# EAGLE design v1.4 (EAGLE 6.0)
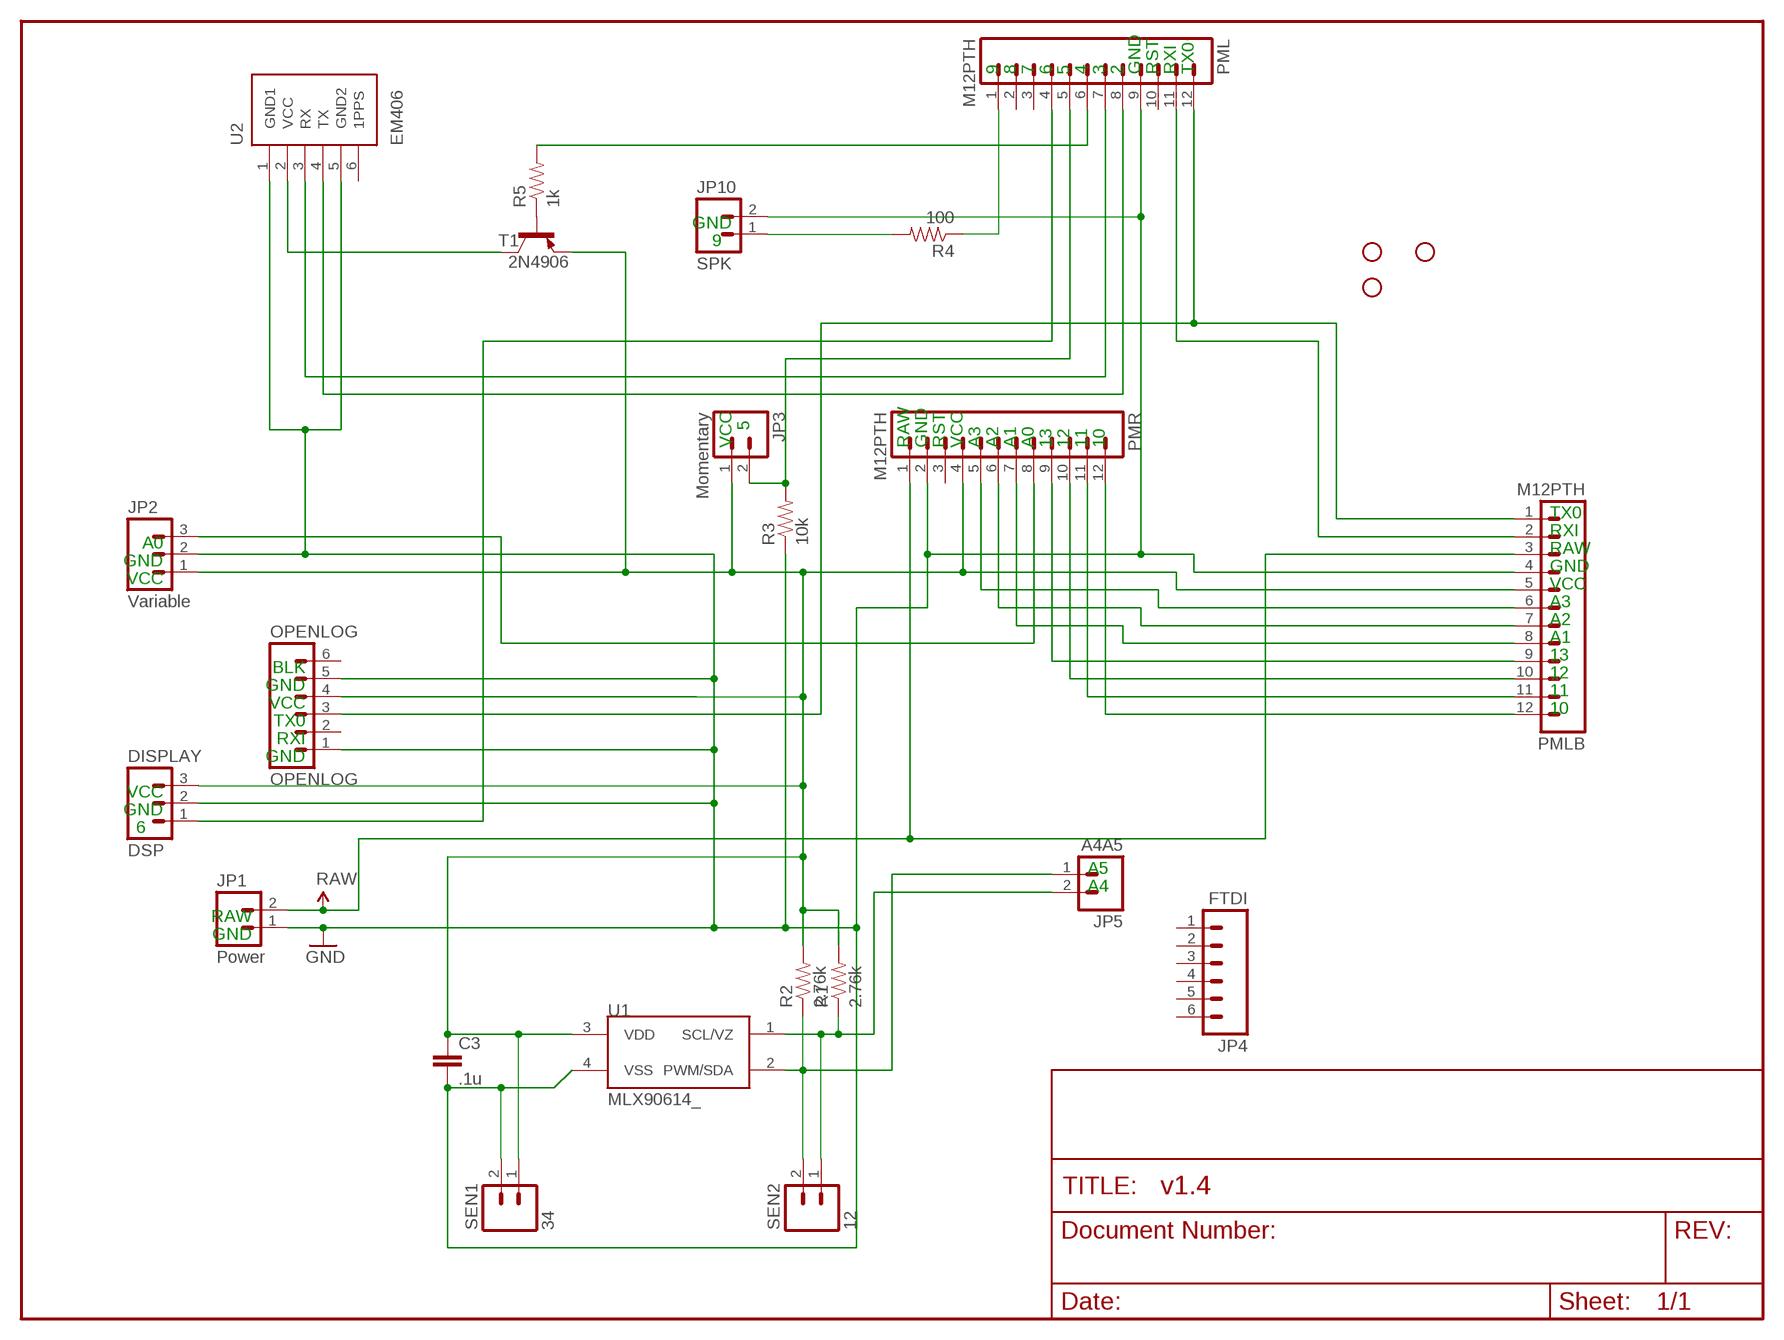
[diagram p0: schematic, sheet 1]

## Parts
2N4906  T1  2N3906-PNP-TO92-EBC  [TO92-EBC]
C3  .1u  CAPPTH1  [CAP-PTH-5MM]
DISPLAY  DSP  M03SCREW_LOCK  [SCREWTERMINAL-3.5MM-3_LOCK.007S]
JP1  Power  M02JST-PTH-2  [JST-2-PTH]
JP2  Variable  M03SCREW_LOCK  [SCREWTERMINAL-3.5MM-3_LOCK.007S]
JP3  Momentary  M02JST-PTH-2  [JST-2-PTH]
JP4  FTDI  M06SIP  [1X06]
JP5  A4A5  M02PTH  [1X02]
JP6  STAND-OFFTIGHT  [STAND-OFF-TIGHT]
JP7  STAND-OFFTIGHT  [STAND-OFF-TIGHT]
JP8  STAND-OFFTIGHT  [STAND-OFF-TIGHT]
JP10  SPK  M02JST-PTH-2  [JST-2-PTH]
OPENLOG  OPENLOG  M06LOCK  [1X06_LOCK]
PML  M12PTH  [1X12]
PMLB  M12PTH  [1X12]
PMR  M12PTH  [1X12]
R1  2.76k  RESISTORPTH-1/4W  [AXIAL-0.4]
R2  2.76k  RESISTORPTH-1/4W  [AXIAL-0.4]
R3  10k  RESISTORPTH-1/4W  [AXIAL-0.4]
R4  100  RESISTORPTH-1/4W  [AXIAL-0.4]
R5  1k  RESISTORPTH-1/4W  [AXIAL-0.4]
SEN1  34  M02JST-PTH-2  [JST-2-PTH]
SEN2  12  M02JST-PTH-2  [JST-2-PTH]
U1  MLX90614_  [TO-39]
U2  EM406  [EM406]

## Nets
GND: C3.2 DISPLAY.2 JP1.1 JP2.2 JP10.2 OPENLOG.1 OPENLOG.5 PML.9 PMLB.4 PMR.2 R3.P$1 SEN1.2 U1.4(VSS) U2.1(GND1) U2.5(GND2)
N$1: JP10.1 R4.P$2
N$2: JP5.1 R2.P$1 SEN2.2 U1.2(PWM/SDA)
N$3: JP3.2 PML.5 R3.P$2
N$4: DISPLAY.1 PML.4
N$5: JP2.3 PMR.8
N$6: OPENLOG.3 PML.12 PMLB.1
N$8: PML.11 PMLB.2
N$9: PMLB.12 PMR.12
N$10: PMLB.11 PMR.11
N$11: PMLB.10 PMR.10
N$12: PMLB.9 PMR.9
N$13: PMLB.8 PMR.7
N$14: PMLB.7 PMR.6
N$15: PMLB.6 PMR.5
N$16: 2N4906.E C3.1 DISPLAY.3 JP2.1 JP3.1 OPENLOG.4 PMLB.5 PMR.4 R1.P$2 R2.P$2 SEN1.1 U1.3(VDD)
N$17: PML.1 R4.P$1
N$18: 2N4906.B R5.P$1
N$19: 2N4906.C U2.2(VCC)
N$20: PML.8 U2.4(TX)
N$21: PML.7 U2.3(RX)
N$22: PML.6 R5.P$2
SENSOR: JP5.2 R1.P$1 SEN2.1 U1.1(SCL/VZ)
VCC: JP1.2 PMLB.3 PMR.1 ; supply symbol labelled RAW
Unconnected: JP4.1 JP4.2 JP4.3 JP4.4 JP4.5 JP4.6 OPENLOG.2 OPENLOG.6 PML.2 PML.3 PML.10 PMR.3 U2.6(1PPS)

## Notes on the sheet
- 9 | 8 | 7 | 6 | 5 | 4 | 3 | 2 | GND | RST | RXI | TX0
- GND
- 9
- 5
- VCC | RAW | GND | RST | VCC | A3 | A2 | A1 | A0 | 13 | 12 | 11 | 10
- TX0
- A0 | RXI
- GND | RAW
- VCC | GND
- VCC
- A3
- A2
- A1
- BLK | 13
- GND | 12
- VCC | 11
- TX0 | 10
- RXI
- GND
- VCC
- GND
- 6
- A5
- A4
- RAW
- GND

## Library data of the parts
2N4906 = transistor-neu-to92:*-PNP-: PNP Transistror
C3 = SparkFun:CAP: Capacitor
DISPLAY JP2 = SparkFun:M03: Header 3 Standard 3-pin 0.1" header. Use with straight break away headers (SKU : PRT-00116), right angle break away headers (PRT-00553), swiss pins (PRT-00743), machine pins (PRT-00117), and female headers (PRT-00115). Molex polarized connector foot print use with SKU : PRT-08232 with associated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
JP1 JP3 JP5 JP10 SEN1 SEN2 = SparkFun:M02: Header 2
JP4 OPENLOG = SparkFun:M06: Header 6 Standard 6-pin 0.1" header. Use with straight break away headers (SKU : PRT-00116), right angle break away headers (PRT-00553), swiss pins (PRT-00743), machine pins (PRT-00117), and female headers (PRT-00115). Molex polarized connector foot print use with SKU : PRT-08094 with associated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
JP6-JP8 = SparkFun:STAND-OFF: Stand Off
PML PMLB PMR = SparkFun:M12: Header 12 Standard 12-pin 0.1" header. Use with straight break away headers (SKU : PRT-00116), right angle break away headers (PRT-00553), swiss pins (PRT-00743), machine pins (PRT-00117), and female headers (PRT-00115).
R1-R5 = SparkFun:RESISTOR: Resistor
U1 = SparkFun:MLX90614: Melexis IR Thermometer
U2 = SparkFun:EM406: EM406 Connector Proven layout and schematic for EM406 connector. Spark Fun Electronics SKU : GPS-00579

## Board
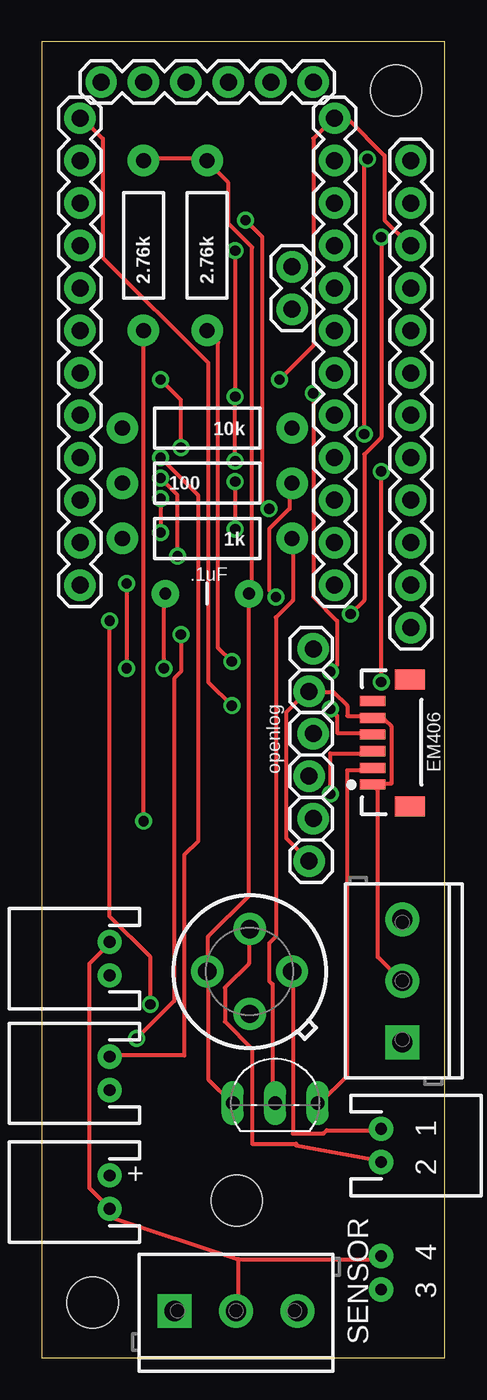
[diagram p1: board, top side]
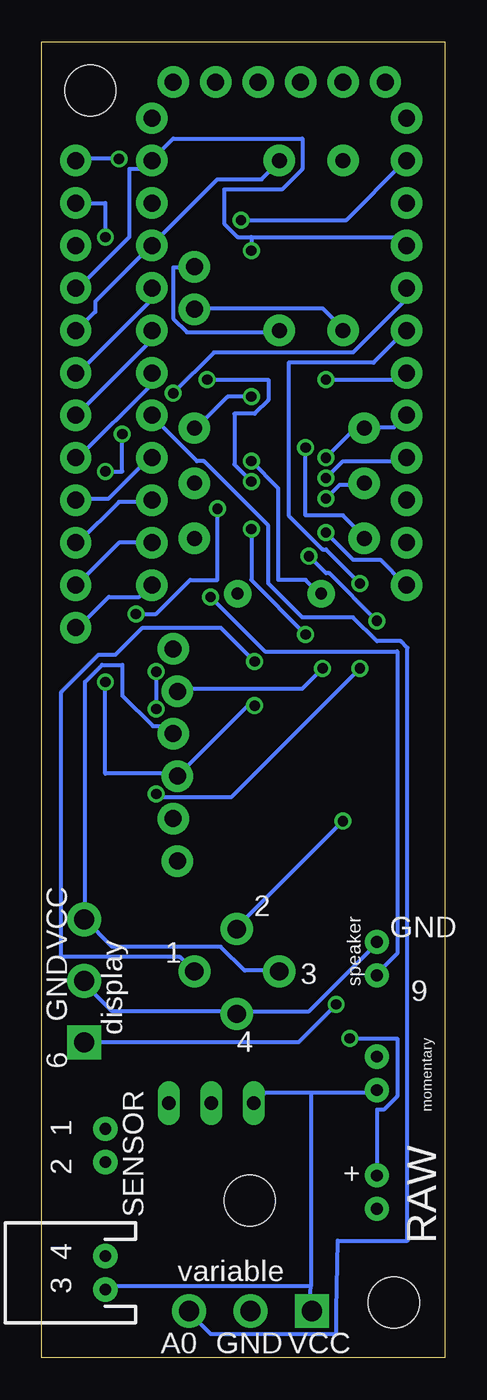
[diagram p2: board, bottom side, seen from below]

Size 24.13 x 78.74 mm. Coordinates in mm from the lower left corner, seen from the top.
Outline: 0,0 24.13,0 24.13,78.74 0,78.74 0,0
Copper layers (1*16): Top 0.035mm / dielectric 1.5mm / Bottom 0.035mm
Design rules: minimum track width 10mil, minimum drill 24mil, track to track 8mil, track to pad 8mil, pad to pad 8mil, via to via 8mil, smd to smd 8mil, copper to edge 40mil, drill to drill 8mil, minimum pad ring 10mil, minimum via ring 8mil, stop-mask expansion 4mil, vias tented up to drill 0mil, thermal gap 10mil

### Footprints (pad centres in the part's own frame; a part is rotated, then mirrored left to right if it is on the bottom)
TO92-EBC = drill 0.813 long: B 0,-1.27; C 2.54,-1.27; E -2.54,-1.27
CAP-PTH-5MM = drill 0.7 pad 1.651: 1 -2.5,0; 2 2.5,0
SCREWTERMINAL-3.5MM-3_LOCK.007S = drill 1.2 pad 2.032 square: 1 -0.178,0 | drill 1.2 pad 2.032: 2 3.5,0; 3 7.178,0
JST-2-PTH = drill 0.7 pad 1.448: 1 -1,0; 2 1,0
1X06 = drill 1.016 pad 1.88: 1 0,0; 2 2.54,0; 3 5.08,0; 4 7.62,0; 5 10.16,0; 6 12.7,0
1X02 = drill 1.016 pad 1.88: 1 0,0; 2 2.54,0
STAND-OFF-TIGHT = hole 3.048: 0,0
1X06_LOCK = drill 1.016 pad 1.88: 1 0,0; 2 2.54,-0.254; 3 5.08,0; 4 7.62,-0.254; 5 10.16,0; 6 12.7,-0.254
1X12 = drill 1.016 pad 1.88: 1 0,0; 2 2.54,0; 3 5.08,0; 4 7.62,0; 5 10.16,0; 6 12.7,0; 7 15.24,0; 8 17.78,0; 9 20.32,0; 10 22.86,0; 11 25.4,0; 12 27.94,0
AXIAL-0.4 = drill 0.9 pad 1.88: P$1 -5.08,0; P$2 5.08,0
TO-39 = drill 1.1 pad 1.93: 1 2.54,0; 2 0,2.54; 3 -2.54,0; 4 0,-2.54
EM406 = smd 0.6 x 1.55: 1 0,0; 2 1,0; 3 2,0; 4 3,0; 5 4,0; 6 5,0 | smd 1.2 x 1.8: P$1 -1.3,-2.225; P$2 6.3,-2.225

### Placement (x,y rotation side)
2N4906  13.97,16.51 0 top
C3  9.91,45.72 180 top
DISPLAY  21.59,19.05 90 top
JP1  4.06,9.91 90 top
JP2  8.13,2.79 0 top
JP3  4.06,17.02 90 top
JP4  16.26,76.33 180 top
JP5  14.99,62.74 90 top
JP6  3.05,3.3 0 top
JP7  21.21,75.82 0 top
JP8  11.68,9.4 90 top
JP10  4.06,23.88 90 top
OPENLOG  16,29.72 90 top
PML  2.29,46.23 90 top
PMLB  22.1,71.63 270 top
PMR  17.53,74.17 270 top
R1  9.91,66.55 90 top
R2  6.1,66.55 90 top
R3  9.91,55.63 180 top
R4  9.91,52.32 0 top
R5  9.91,49.02 180 top
SEN1  20.32,5.08 90 bottom
SEN2  20.32,12.7 270 top
U1  12.45,23.11 0 top
U2  19.81,34.29 90 top

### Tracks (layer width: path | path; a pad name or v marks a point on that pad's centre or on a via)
GND  (via drill 0.61)
  Top 0.254: v11.58,66.24 v11.58,57.51 v11.58,53.65 | v7.32,41.25 7.32,45.72 C3.2 | OPENLOG.1 14.63,31.09 14.63,38.61 15.85,39.83 OPENLOG.5 16.05,39.83 17.48,39.83 18.29,39.01 18.29,38.41 19.71,38.41 U2.5 19.91,38.2 20.52,38.2 20.93,37.8 20.93,34.34 19.91,34.34 U2.1 19.91,34.14 20.12,33.93 20.12,23.98 21.54,22.55 DISPLAY.2 | JP10.2 4.06,24.79 2.85,23.57 2.85,10.16 4.06,8.94 JP1.1 4.06,8.43 11.79,5.89 | 11.79,5.89 20.32,5.89 SEN1.2 | 11.79,5.89 11.79,2.85 JP2.2
  Bottom 0.254: 11.58,67.06 12.39,67.06 13.21,67.87 13.21,69.9 9.75,69.9 8.53,71.12 8.53,72.95 16.26,72.95 17.48,71.73 PMR.2 17.68,71.53 18.09,71.12 18.9,71.12 18.9,67.06 21.95,64.01 PMLB.4 | 11.58,67.06 2.85,67.06 2.44,66.65 PML.9 | v11.58,57.51 13.01,57.51 14.83,55.68 R3.P$1 | 11.58,67.06 v11.58,66.24 | v7.32,41.25 8.53,40.03 15.85,40.03 OPENLOG.5 | JP10.2 4.06,24.79 8.13,20.73 12.39,20.73 U1.4 12.6,20.73 19.91,20.73 21.54,22.35 DISPLAY.2 | v11.58,53.65 9.96,52.02 9.96,46.53 8.33,46.53 7.52,45.72 C3.2
N$1  (via drill 0.61)
  Top 0.254: v14.02,45.52 13.61,45.92 13.61,49.58 14.83,50.8 14.83,52.22 R4.P$2
  Bottom 0.254: v14.02,45.52 10.77,42.27 2.85,42.27 2.85,24.18 4.06,22.96 JP10.1
N$2  (via drill 0.61)
  Top 0.254: v6.1,32.11 R2.P$1 | SEN2.2 20.32,11.79 15.24,12.7 15.24,12.8 12.6,12.8 12.6,18.49 10.97,20.12 10.97,22.15 12.39,23.57 12.39,25.6 U1.2
  Bottom 0.254: R2.P$1 6.1,61.57 7.32,62.79 14.83,62.79 JP5.1 | v6.1,32.11 12.39,25.81 U1.2
N$3  (via drill 0.61)
  Top 0.254: v7.11,53.85 9.35,51.61 9.35,30.89 8.53,30.07 8.53,18.09 4.06,18.09 JP3.2
  Bottom 0.254: v7.11,53.85 5.49,55.47 4.88,55.47 R3.P$2 4.67,55.68 3.05,55.68 2.44,56.29 PML.5
N$4  (via drill 0.61)
  Top 0.254: v7.11,52.63 8.13,51.61 v8.13,47.95 | v4.06,44.09 4.06,26.42 6.5,23.98 v6.5,21.13
  Bottom 0.254: v7.11,52.63 6.1,53.65 2.64,53.65 2.44,53.85 PML.4 | v8.13,47.95 7.11,46.94 6.91,46.94 v4.06,44.09 | v6.5,21.13 8.74,18.9 21.54,18.9 DISPLAY.1
N$5
  Bottom 0.254: PMR.8 17.48,56.29 14.83,53.65 14.43,53.65 10.57,49.78 10.57,46.33 8.53,44.3 5.49,44.3 4.06,42.88 2.64,42.88 2.23,42.47 2.23,7.01 6.4,7.01 6.5,2.85 6.5,1.42 14.02,1.42 15.24,2.64 JP2.3
N$6  (via drill 0.61)
  Top 0.254: v11.38,39.01 9.96,40.44 9.96,59.54 3.66,65.84 3.66,72.95 2.44,74.17 PML.12 | v19.51,71.73 19.3,71.53 v19.3,55.27 | v20.32,40.44 v20.32,53.03
  Bottom 0.254: v11.38,39.01 11.79,39.01 OPENLOG.3 16.05,34.95 20.32,34.95 v20.32,40.44 | v19.51,71.73 21.95,71.73 PMLB.1 | v19.3,55.27 19.3,53.03 v20.32,53.03
N$8  (via drill 0.61)
  Top 0.254: v12.19,68.07 13.21,67.06 13.21,51.21 v13.61,50.8 | v18.49,44.5 19.3,45.31 19.3,54.05 20.32,55.07 v20.32,67.06
  Bottom 0.254: v12.19,68.07 5.89,68.07 2.44,71.53 PML.11 | v13.61,50.8 13.61,46.53 15.24,46.53 17.27,44.5 v18.49,44.5 | v20.32,67.06 20.32,69.09 PMLB.2
N$9
  Bottom 0.254: PMR.12 17.68,46.13 18.29,45.52 20.12,45.52 21.95,43.69 PMLB.12
N$10
  Bottom 0.254: PMR.11 19.51,48.77 21.95,46.33 PMLB.11
N$11
  Bottom 0.254: PMLB.10 21.95,48.77 19.51,51.21 17.68,51.21 PMR.10
N$12
  Bottom 0.254: PMR.9 17.68,53.85 20.12,51.41 21.95,51.41 PMLB.9
N$13
  Bottom 0.254: PMLB.8 21.95,53.85 17.68,58.12 17.68,58.93 PMR.7
N$14
  Bottom 0.254: PMLB.7 21.95,56.49 17.68,60.76 17.68,61.37 PMR.6
N$15
  Bottom 0.254: PMLB.6 21.95,58.93 17.68,63.2 17.68,64.01 PMR.5
N$16
  Top 0.254: R2.P$2 6.1,71.73 9.75,71.73 R1.P$2 9.96,71.53 11.18,70.31 11.18,67.87 12.6,66.45 12.6,45.72 C3.1 12.39,45.72 12.39,27.64 9.96,25.2 9.96,23.16 U1.3 9.96,22.96 9.96,16.66 11.38,15.24 2N4906.E
  Bottom 0.254: PMLB.5 21.95,61.57 20.93,62.59 20.93,63.2 17.68,66.45 PMR.4 17.48,66.65 13.61,70.51 10.97,70.51 9.96,71.53 R1.P$2 | OPENLOG.4 16.26,37.39 16.66,37.8 17.48,37.8 19.3,39.62 19.3,41.45 20.52,41.45 21.54,40.44 21.54,26.42 DISPLAY.3 21.54,26.21 19.91,24.59 13.41,24.59 11.99,23.16 9.96,23.16 U1.3 | 8.03,4.27 20.32,4.27 SEN1.1 | 8.03,4.27 8.13,2.85 JP2.1 | 8.03,15.85 4.06,15.85 JP3.1 | 8.03,15.85 10.77,15.85 11.38,15.24 2N4906.E | 8.03,15.85 8.03,4.27
N$17  (via drill 0.61)
  Top 0.254: v7.11,51.41 v7.11,49.38
  Bottom 0.254: v7.11,49.38 5.49,47.75 3.86,47.75 2.44,46.33 PML.1 | v7.11,51.41 6.3,52.22 4.88,52.22 R4.P$1
N$18
  Top 0.254: 2N4906.B 13.82,15.24 13.82,22.35 13.61,22.55 13.61,24.79 14.02,25.2 14.02,44.3 15.04,45.31 15.04,48.97 R5.P$1
N$19
  Top 0.254: U2.2 19.71,35.15 18.29,35.15 18.29,16.87 16.66,15.24 2N4906.C
N$20  (via drill 0.61)
  Top 0.254: v17.27,38.81 17.68,38.41 17.68,37.39 19.71,37.39 U2.4 | v17.27,41.05 17.68,41.45 17.68,44.09 16.26,45.52 v16.26,57.71
  Bottom 0.254: v17.27,41.05 v17.27,38.81 | v16.26,57.71 13.82,60.15 5.49,60.15 2.44,63.2 2.44,64.01 PML.8
N$21  (via drill 0.61)
  Top 0.254: v17.27,33.73 17.27,36.17 19.71,36.17 U2.3 | v5.08,46.33 v5.08,41.25
  Bottom 0.254: v17.27,33.73 17.07,33.53 12.8,33.53 v5.08,41.25 | v5.08,46.33 7.11,48.36 7.32,48.36 9.35,50.39 9.35,59.54 4.27,59.54 2.44,61.37 PML.7
N$22  (via drill 0.61)
  Top 0.254: v7.11,58.52 8.33,57.3 v8.33,54.46
  Bottom 0.254: v7.11,58.52 2.85,58.52 2.44,58.93 PML.6 | v8.33,54.46 8.33,50.39 6.1,50.39 4.88,49.17 R5.P$2
SENSOR  (via drill 0.61)
  Top 0.254: SEN2.1 20.32,13.61 17.07,13.61 16.87,13.41 15.04,13.41 15.04,22.96 U1.1 | v11.38,41.66 10.57,42.47 10.57,60.76 9.96,61.37 R1.P$1
  Bottom 0.254: R1.P$1 9.96,61.37 15.44,61.37 16.26,62.18 16.26,65.23 15.04,65.23 JP5.2 | v11.38,41.66 13.41,43.69 18.09,43.69 19.71,42.06 20.73,42.06 22.96,39.83 22.96,23.98 15.85,23.98 U1.1
VCC  (via drill 0.61)
  Top 0.254: v5.69,19.1 7.92,21.34 7.92,40.64 8.33,41.05 v8.33,43.28 | v11.58,52.43 v11.58,49.58 | v14.22,58.52 16.26,60.55 16.26,72.95 17.48,74.17 PMR.1 18.29,74.17 20.52,71.93 20.52,68.07 21.95,66.65 PMLB.3
  Bottom 0.254: JP1.2 4.06,14.83 3.66,14.83 2.85,15.65 2.85,19.1 v5.69,19.1 | v8.33,43.28 11.58,46.53 v11.58,49.58 | v11.58,52.43 12.6,53.44 12.6,56.49 11.38,56.49 10.57,57.3 10.57,58.52 v14.22,58.52

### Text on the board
tPlace: .1uF | openlog | EM406 | 1 | 2 | + | SENSOR | 4 | 3
bPlace: VCC | speaker | 2 | GND | 1 | GND | 3 | 9 | display | 4 | 6 | SENSOR | momentary | 1 | RAW | 2 | + | 4 | variable | 3 | VCC | GND | A0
